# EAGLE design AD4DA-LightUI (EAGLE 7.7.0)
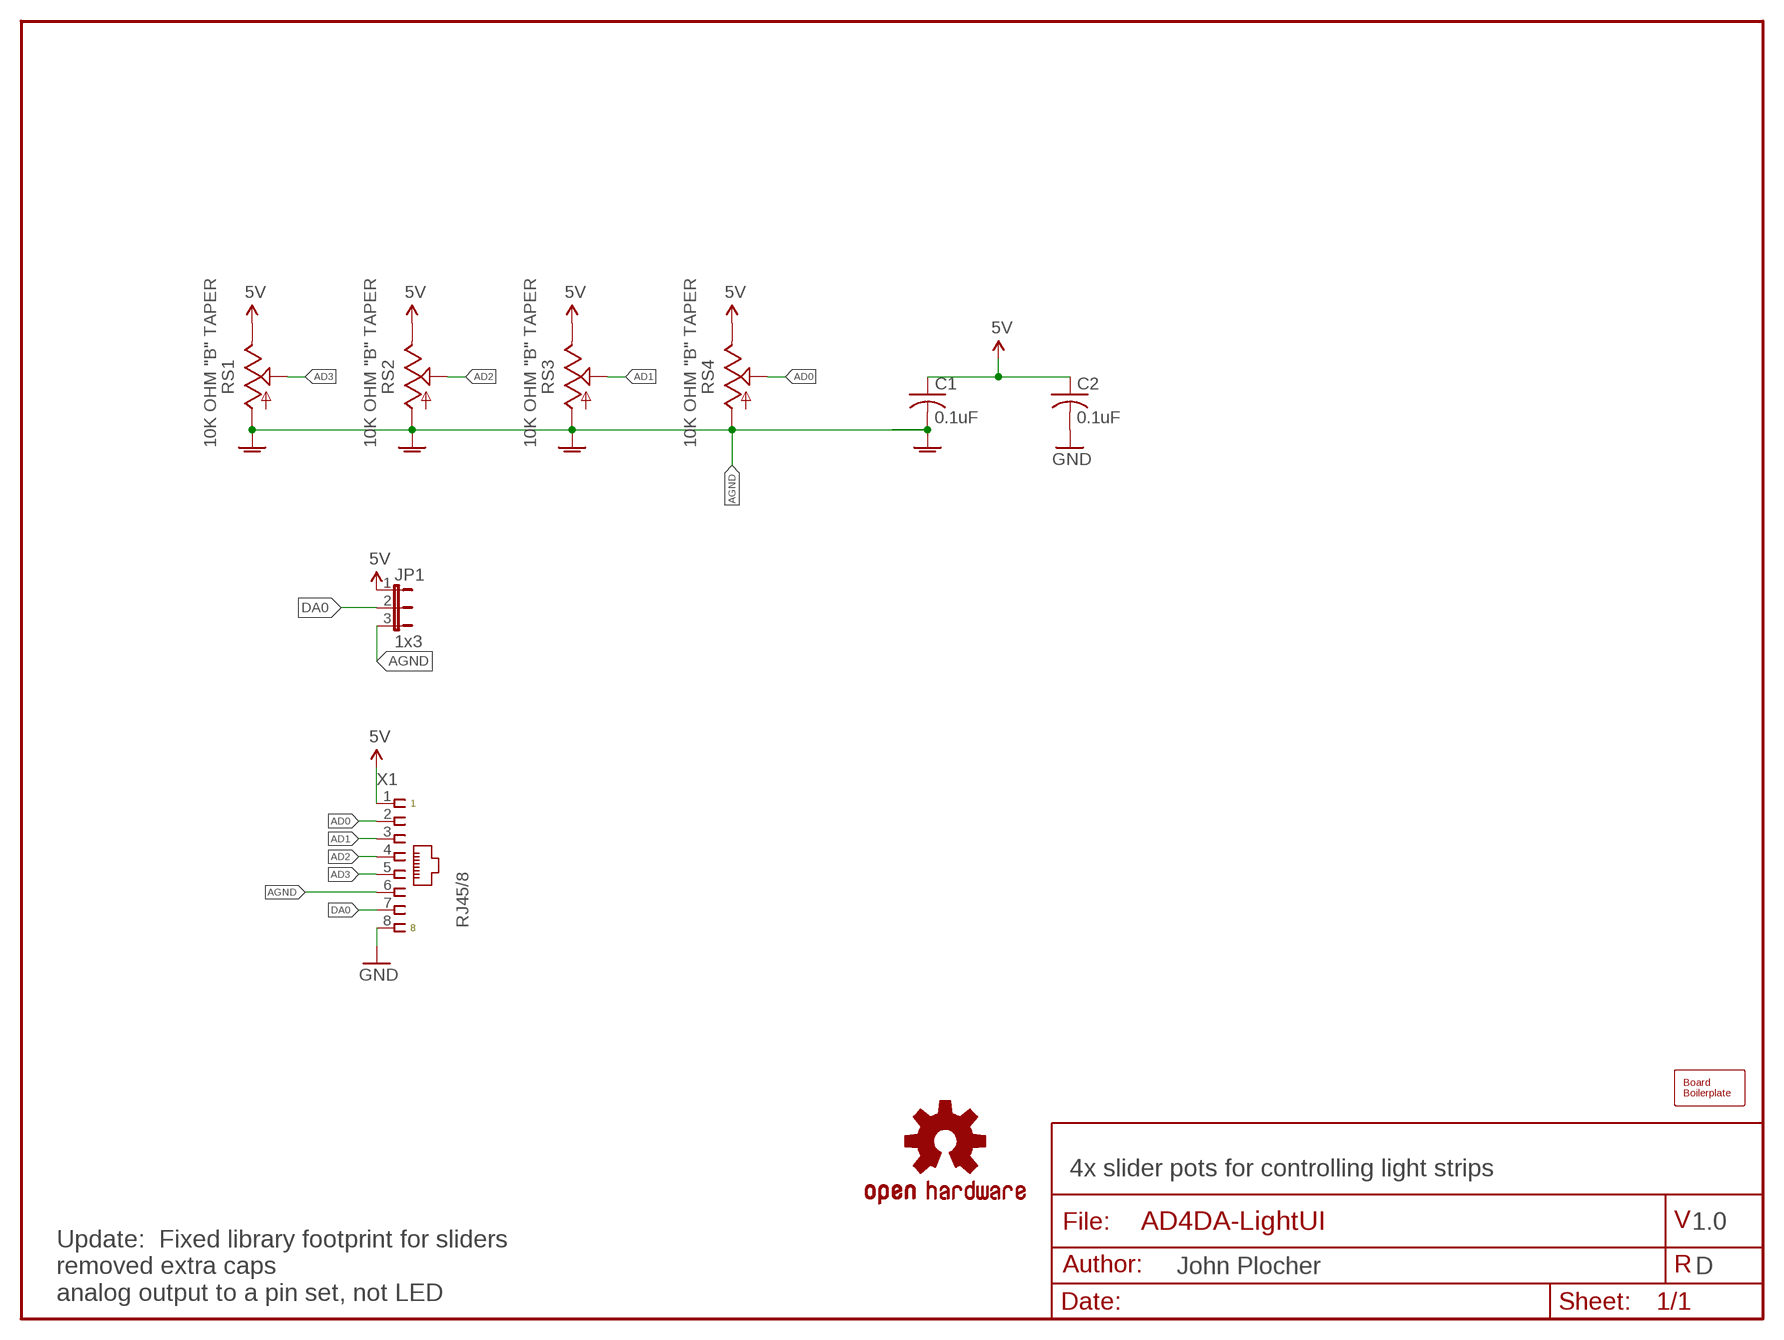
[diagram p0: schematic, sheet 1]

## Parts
BOARD1  10x7cm  BOARD80X70  [BOARD-DINRAIL-3.17INX7CM]
C1  0.1uF  CAPPTH1  [C050-024X044]
C2  0.1uF  CAPPTH1  [C050-024X044]
JP1  1x3  JUMPER-3PTH-LOCK  [1X03]
LOGO1  DOC-OSHW-LOGO-L  [OSHW-LOGO-L]
RS1  10K OHM "B" TAPER  R-SLIDE-POT-45MM  [SLIDER-45MM]
RS2  10K OHM "B" TAPER  R-SLIDE-POT-45MM  [SLIDER-45MM]
RS3  10K OHM "B" TAPER  R-SLIDE-POT-45MM  [SLIDER-45MM]
RS4  10K OHM "B" TAPER  R-SLIDE-POT-45MM  [SLIDER-45MM]
X1  RJ45/8  CONNECTOR-RJ45-FRONT  [RJ45-NO-SHIELD]

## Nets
5V: C1.1 C2.1 JP1.1 RS1.E RS2.E RS3.E RS4.E X1.1
AD0: RS4.S X1.2
AD1: RS3.S X1.3
AD2: RS2.S X1.4
AD3: RS1.S X1.5
AGND: C1.2 JP1.3 RS1.A RS1.AGND@0(AGND) RS1.AGND@1(AGND) RS2.A RS2.AGND@0(AGND) RS2.AGND@1(AGND) RS3.A RS3.AGND@0(AGND) RS3.AGND@1(AGND) RS4.A RS4.AGND@0(AGND) RS4.AGND@1(AGND) X1.6
DA0: JP1.2 X1.7
GND: C2.2 X1.8

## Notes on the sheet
- 4x slider pots for controlling light strips
- 1.0
- D
- Update:  Fixed library footprint for sliders
  removed extra caps
  analog output to a pin set, not LED

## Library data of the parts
BOARD1 = SPCoast:BOARD
C1 C2 = SPCoast:CAP*
JP1 = SPCoast:JUMPER-3
LOGO1 = SPCoast:DOC-OSHW-LOGO-: Open Source Hardware Logo
RS1-RS4 = SPCoast:R-SLIDE-POT: Slide-type potentiometer- COM-9119
X1 = SPCoast:CONNECTOR-RJ45: Tyco CORCOM Modular RJ Jacks No Shield; AMP: 520151-4; OPL: none

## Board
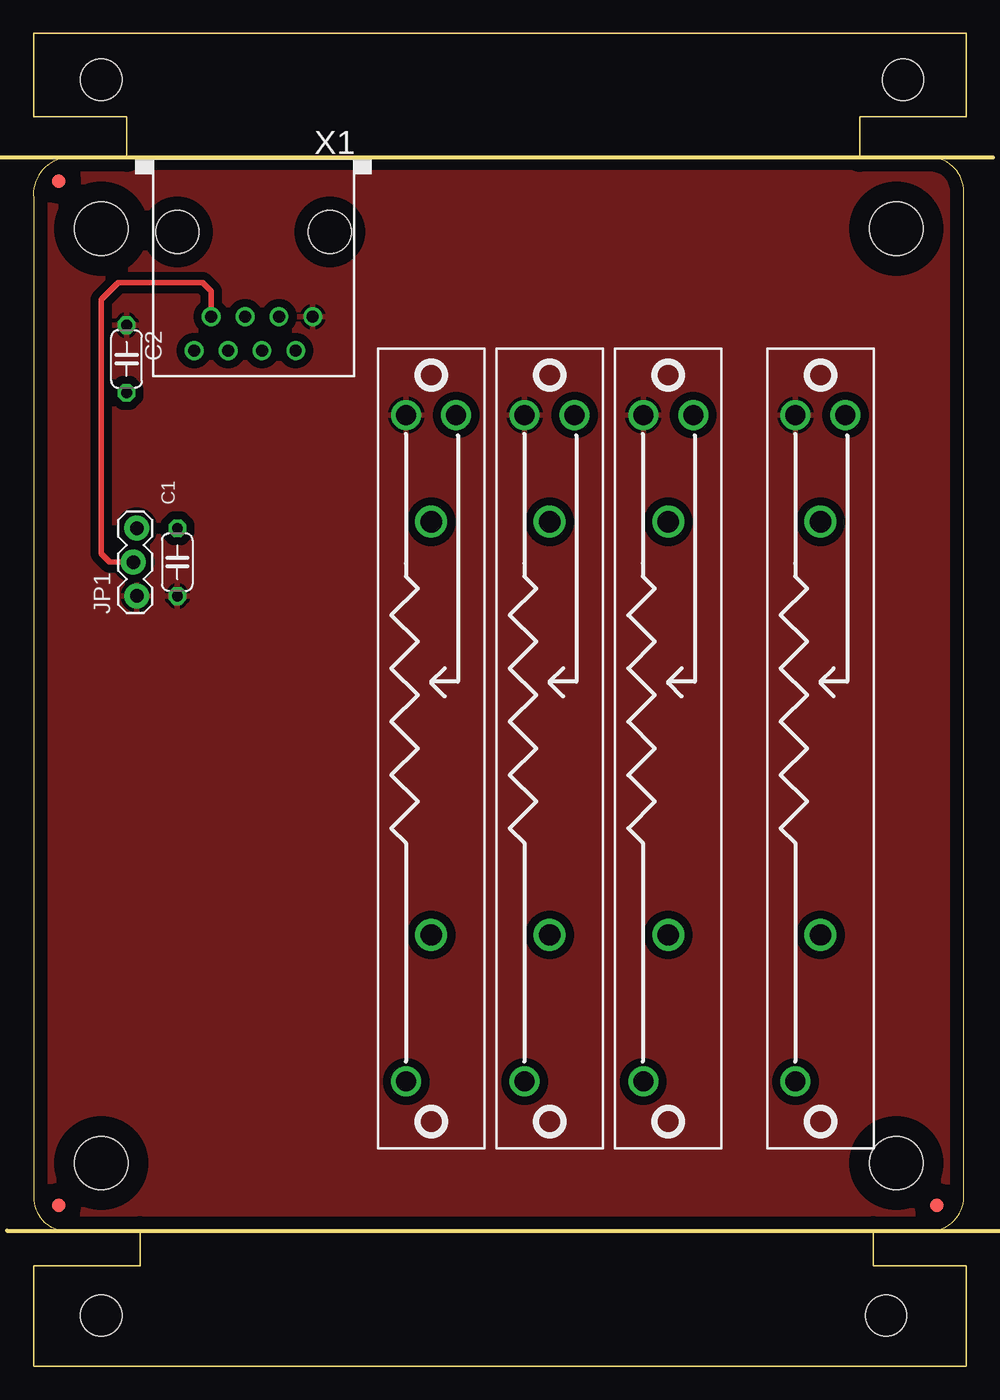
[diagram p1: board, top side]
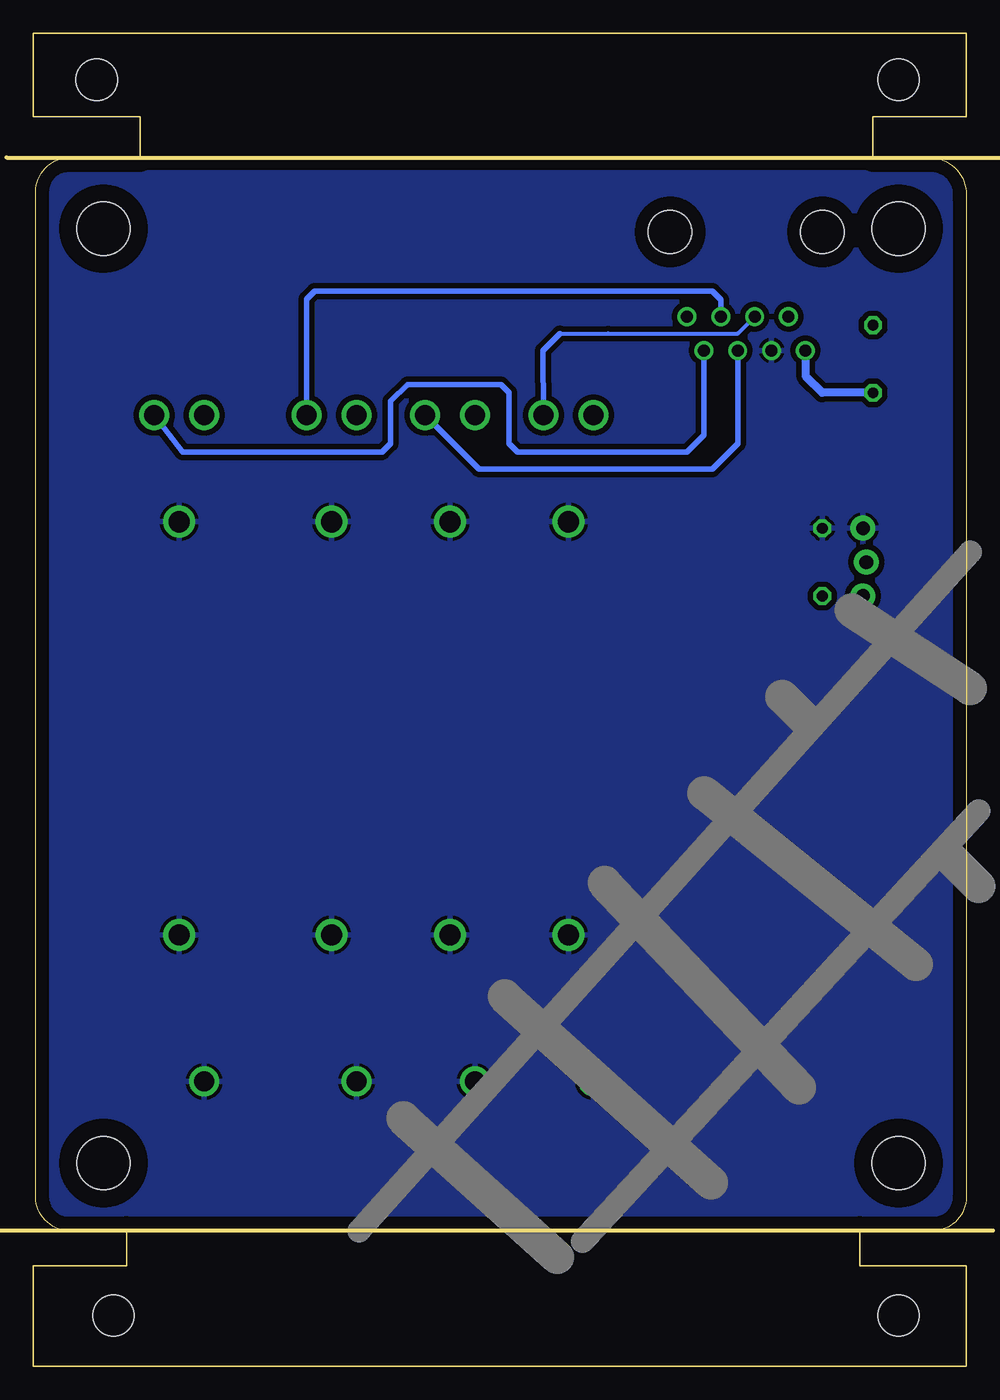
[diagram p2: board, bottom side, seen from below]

Size 70.01 x 100 mm. Coordinates in mm from the lower left corner, seen from the top.
Copper layers (1*16): Top 0.035mm / dielectric 1.5mm / Bottom 0.035mm
Design rules "default": minimum track width 10mil, minimum drill 0.6mm, track to track 8mil, track to pad 8mil, pad to pad 8mil, via to via 8mil, smd to smd 8mil, copper to edge 40mil, drill to drill 8mil, minimum pad ring 10mil, minimum via ring 8mil, stop-mask expansion 4mil, vias tented up to drill 0mil, thermal gap 10mil

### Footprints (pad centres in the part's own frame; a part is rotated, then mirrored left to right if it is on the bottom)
BOARD-DINRAIL-3.17INX7CM = smd 1 x 1: 1 1.905,12.065; 2 67.79,12.065; 3 1.905,88.9 | hole 4: 64.742,15.24; 5.08,85.344; 64.742,85.344; 5.08,15.24 | hole 3.1: 5.08,96.52; 65.25,96.52; 5.08,3.81; 63.98,3.81
C050-024X044 = drill 0.813 octagon: 1 -2.54,0; 2 2.54,0
1X03 = drill 1.016 pad 1.88: 1 0,-0.127; 2 2.54,0.127; 3 5.08,-0.127
SLIDER-45MM = drill 1.5: A 25,-1.875; E -25,-1.875; S -25,1.875 | drill 1.6: AGND@0 -17,0; AGND@1 14,0
RJ45-NO-SHIELD = drill 0.9 pad 1.4: 1 -4.445,6.35; 2 -3.175,8.89; 3 -1.905,6.35; 4 -0.635,8.89; 5 0.635,6.35; 6 1.905,8.89; 7 3.175,6.35; 8 4.445,8.89 | hole 3.251: -5.715,0; 5.715,0

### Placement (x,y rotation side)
BOARD1  0.01,0 0 top
C1  10.81,60.33 90 top
C2  7,75.56 270 top
JP1  7.63,57.78 90 top
LOGO1  5.09,15.24 0 top
RS1  29.86,46.35 270 top
RS2  38.75,46.35 270 top
RS3  47.64,46.35 270 top
RS4  59.07,46.35 270 top
X1  16.52,85.09 180 top

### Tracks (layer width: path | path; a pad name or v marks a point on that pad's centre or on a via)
5V
  pour Top (isolate 0.61): 0.01,89.53 69.86,89.53 69.86,11.43 0.01,11.43
AD0
  Bottom 0.406: RS4.S 58.8,68.58 43.83,68.58 43.19,69.22 43.19,72.39 41.92,73.66 34.94,73.66 34.3,73.03 34.3,69.22 33.67,68.58 20.97,68.58 19.7,69.85 X1.2
AD1
  Bottom 0.406: X1.3 18.43,80.01 19.06,80.64 20.33,80.64 48.91,80.64 49.51,80.04 RS3.S
AD2
  Bottom 0.406: RS2.S 36.58,67.31 19.06,67.31 17.16,69.22 X1.4
AD3
  Bottom 0.305: 30.49,77.47 26.89,77.47 17.16,77.47 X1.5
  Bottom 0.406: RS1.S 31.76,76.2 30.49,77.47
AGND
  pour Bottom (isolate 0.406): 0.01,89.53 69.86,89.53 69.86,11.43 0.01,11.43
  pour Bottom: 25.41,19.05 62.24,19.05 62.24,66.04 27.95,66.04 25.41,66.04
DA0
  Top 0.406: JP1.2 5.73,60.33 5.09,60.96 5.09,80.01 6.36,81.28 12.71,81.28 13.35,80.64 X1.7
GND
  Bottom 0.61: X1.8 12.08,74.3 10.81,73.03 C2.2

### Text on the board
tDocu: v1.0D | R G B | W | AD3 | AD2 | AD1 | AD0 | DA0 | AD3 | AD2 | AD1 | AD0 | +5 | Dgnd | Agnd | LightUI | Agnd | DA0 | +5 | D/A out | 2018-07 | OSHW / John Plocher | LightUI | v1.0D
bDocu: Made in the PCR, Coast Division, NMRA | LightUI | Solder Side | Go Bears! | Model Railroading is fun! | www . SPCoast . com
Changes: Added Carrier template, shrunk board size

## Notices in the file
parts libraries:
SparkFun-Aesthetics: Licensing: CC v3.0 Share-Alike You are welcome to use this library for commercial purposes.
SPCoast: http://freedomdefined.org/OSHW Creative Commons - Attribution - ShareAlike 3.0
